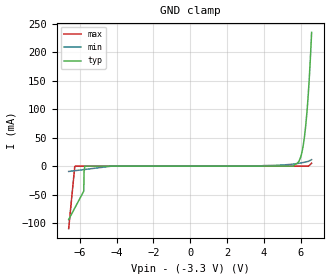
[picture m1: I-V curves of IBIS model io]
|Texas Instruments Incorporated
| 1 Channel ESD Protection Diode for High Speed Data Lines up to 20Gbps
| Marketing part#   Digital Voltage Range   Package-type   #pins
| TPD1E01B04DPLR   -3.6V-3.6V   X1SON   2
| TPD1E01B04DPYR   -3.6V-3.6V   X1SON   2
[IBIS Ver]   4.1
[File name]   tpd1e01b04.ibs
[File Rev]   1.0
[Date]   05/20/2016
[Source]
| Texas Instruments Incorporated.
| Analog-eLab Design Center, HPA
| 12500 TI Blvd
| Dallas, TX -75243
[Notes]   Revision History:
| Rev 1.0: 05/20/2016
| - Initial version of the model
| - Model generated from bench data
| - Model matched to SPICE simulation
| - C_comp although listed in numerical order of value are
|   obtained from varying PVT conditions. For PVT conditions for
|   each specific value refer the buffer description under
|   respective [Model]. IBIS model user is responsible for using
|   appropriate C_comp to simulate for Signal Integrity.
[Disclaimer]
| This model is designed as an aid for customers of Texas Instruments.
| TI and its licensors and suppliers make no warranties, either expressed
| or implied, with respect to this  model, including the warranties of
| merchantability or fitness for a particular purpose. The model is
| provided solely on an "as is" basis. The entire risk as to its quality
| and performance is with the customer.
[Copyright]
(C) Copyright 2016 Texas Instruments Incorporated.All rights reserved.
|   TPD1E01B04DPL
[Component]   TPD1E01B04DPL
[Manufacturer]   TI
[Package]   |2 X2SON - DPL package
|   typ   min   max
R_pkg   1.000e-200   1.000e-200   1.000e-200
L_pkg   1.000e-200   1.000e-200   1.000e-200
C_pkg   1.000e-200   1.000e-200   1.000e-200
[Pin]  signal_name   model_name   R_pin   L_pin   C_pin
1   1   io   4.000E-02  3.000E-10  1.000E-14
2   2   gnd   1.000e-200 1.000e-200 1.000e-200
|   TPD1E01B04DPY
[Component]   TPD1E01B04DPY
[Manufacturer]   TI
[Package]   |2 X1SON - DPY package
|   typ   min   max
R_pkg   1.000e-200   1.000e-200   1.000e-200
L_pkg   1.000e-200   1.000e-200   1.000e-200
C_pkg   1.000e-200   1.000e-200   1.000e-200
[Pin]  signal_name   model_name   R_pin   L_pin   C_pin
1   1   io   4.000E-02   6.000E-10   2.000E-14
2   2   gnd   1.000e-200  1.000e-200  1.000e-200
| Models and submodels in the file (1): io (Terminator)
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|   io Model
[Model]   io
Model_type   Terminator
|   typ   min   max
C_comp   1.700E-13   1.501E-13   1.999E-13
| Where nom  PVT is Nominal Process, 3.3V, 25C
|   Fast PVT is Strong Process,  3.0V, -40C
|   Slow PVT is Weak Process,   3.6V, 125C
[Voltage Range]   6.6   6.0   7.2
[Temperature Range]   25   125   -40
[Power Clamp Reference]   3.3   3.0   3.6
[GND Clamp Reference]   -3.3   -3.0   -3.6
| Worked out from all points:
|   GND clamp passes 1 mA (typ) near -5.72 V on its own axis
[GND Clamp]
|   Voltage   I(typ)   I(min)   I(max)
-6.6V     -94mA      -9.4mA     -110mA
-6.27V    -73.85mA   -8.078mA   -1mA
-6.237V   -71.83mA   -7.946mA   -1.059nA
-5.78V    -43.97mA   -6.119mA   -740.4pA
-5.765V   -10mA      -6.059mA   -731.7pA
-5.721V   -1.226nA   -5.882mA   -706.9pA
5.632V    1.213nA    3.759mA    589.6pA
5.972V    12.86mA    5.35mA     816.3pA
6.204V    49.45mA    6.77mA     1.019nA
6.402V    118.2mA    8.243mA    1.229nA
6.534V    190.1mA    10.25mA    3mA
6.6V      235.2mA    11.4mA     5mA
[Power Clamp]
|   Voltage   I(typ)   I(min)   I(max)
-6.6V     0A         0A         0A
0V        0A         0A         0A
13.2V     0A         0A         0A
